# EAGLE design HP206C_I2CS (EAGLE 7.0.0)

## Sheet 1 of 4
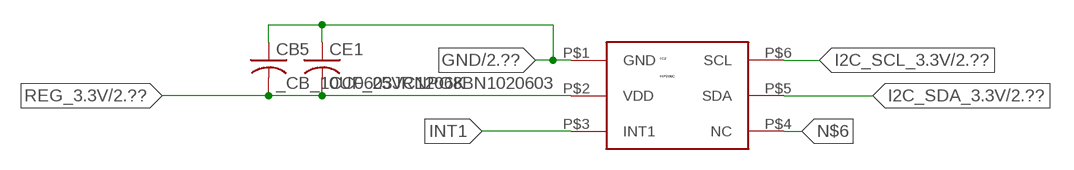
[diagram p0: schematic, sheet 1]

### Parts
CB5  _CB_10UF_25VC1206K  [_CB_10UF_25V]
CE1  CC0603JRNPO8BN1020603  [CC0603JRNPO8BN102]
IC2  HP206C  [HP206C]

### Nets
GND: CB5.1 CE1.1 IC2.P$1(GND) ; also sheet 2,4
I2C_SCL_3.3V: IC2.P$6(SCL) ; also sheet 2
I2C_SDA_3.3V: IC2.P$5(SDA) ; also sheet 2
INT1: IC2.P$3(INT1)
N$6: IC2.P$4(NC)
REG_3.3V: CB5.2 CE1.2 IC2.P$2(VDD) ; also sheet 2

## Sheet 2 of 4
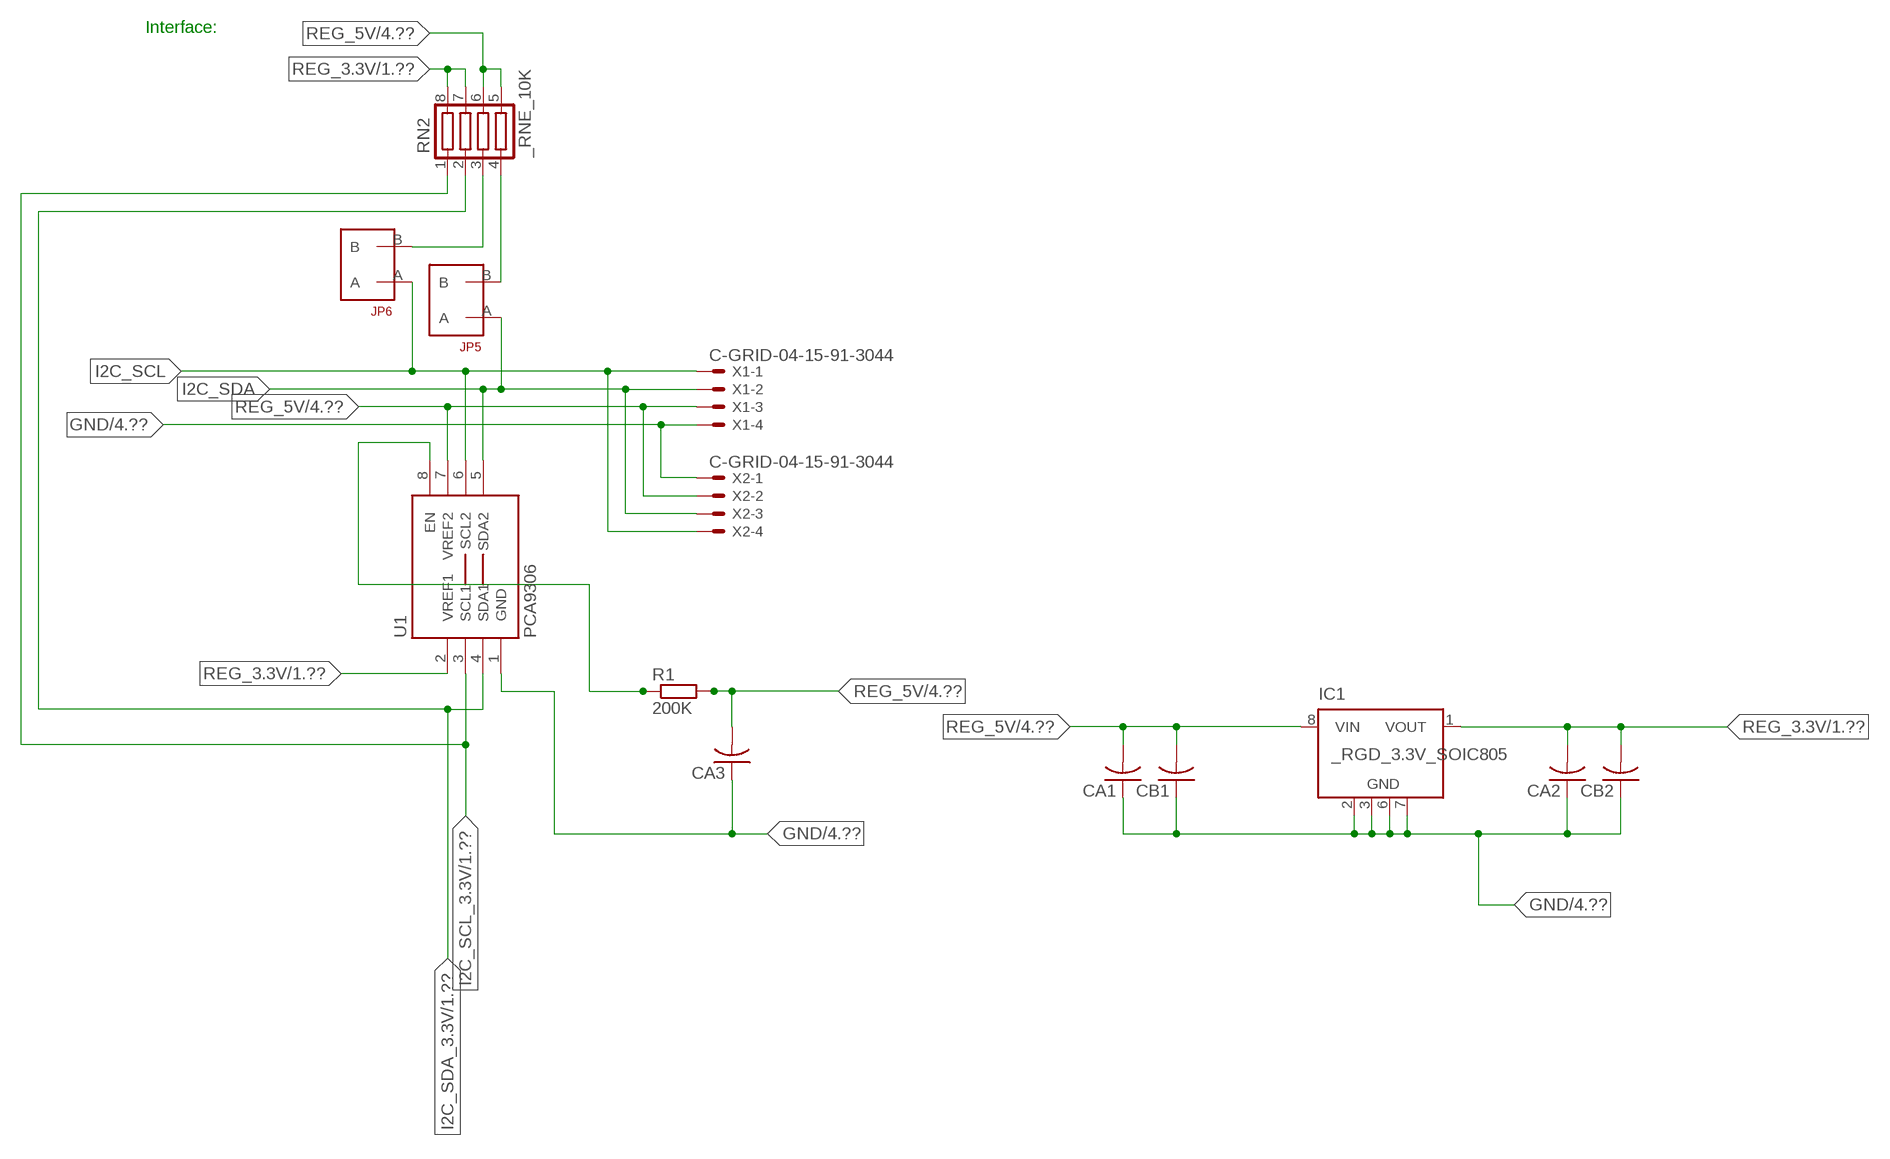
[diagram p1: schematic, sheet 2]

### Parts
CA1  CC1206KRX7R9BB104  [.1UF]
CA2  CC1206KRX7R9BB104  [.1UF]
CA3  CC1206KRX7R9BB104  [.1UF]
CB1  TMK316F106ZL-TC1206K  [TMK316F106ZL-T]
CB2  TMK316F106ZL-TC1206K  [TMK316F106ZL-T]
IC1  _RGD_3.3V_SOIC805  [_RGC_3.3V_SOIC8]
JP5  JUMPER_1X2_2MM  [JUMPER_1X2_2MM]
JP6  JUMPER_1X2_2MM  [JUMPER_1X2_2MM]
R1  200K  RESISTOR_SMT-0603  [R603]
RN2  _RNE_10K  [RNE]
U1  PCA9306  PCA9306_NCD  [PSOP-8]
X1  C-GRID-04-15-91-3044  [15-91-04]
X2  C-GRID-04-15-91-3044  [15-91-04]

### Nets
GND: CA1.1 CA2.1 CA3.1 CB1.1 CB2.1 IC1.2(GND) IC1.3(GND) IC1.6(GND) IC1.7(GND) U1.1(GND) X1.4 X2.1 ; also sheet 1,4
I2C_SCL: JP6.A U1.6(SCL2) X1.1 X2.4
I2C_SCL_3.3V: RN2.1 U1.3(SCL1) ; also sheet 1
I2C_SDA: JP5.A U1.5(SDA2) X1.2 X2.3
I2C_SDA_3.3V: RN2.2 U1.4(SDA1) ; also sheet 1
N$1: JP6.B RN2.3
N$2: JP5.B RN2.4
N$3: R1.1 U1.8(EN)
REG_3.3V: CA2.2 CB2.2 IC1.1(VOUT) RN2.7 RN2.8 U1.2(VREF1) ; also sheet 1
REG_5V: CA1.2 CA3.2 CB1.2 IC1.8(VIN) R1.2 RN2.5 RN2.6 U1.7(VREF2) X1.3 X2.2 ; also sheet 4
Unconnected: IC1.4(NC) IC1.5(NC)

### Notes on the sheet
- Interface:

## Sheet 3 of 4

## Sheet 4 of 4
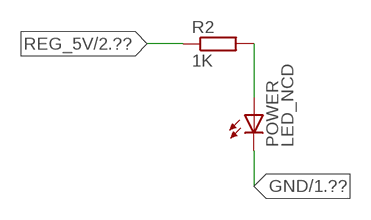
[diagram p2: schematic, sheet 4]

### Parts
POWER  LED_NCD  [CHIPLED_0603]
R2  1K  RESISTOR_SMT-0402  [R402]

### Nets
GND: POWER.C ; also sheet 1,2
N$4: POWER.A R2.2
REG_5V: R2.1 ; also sheet 2

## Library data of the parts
CA1-CA3 = NCD_ULTIMATE_LIBRARY:CC1206KRX7R9BB104: Capacitor CA .1uF 50V SMT C1206K CC1206KRX7R9BB104
CB1 CB2 = NCD_ULTIMATE_LIBRARY:TMK316F106ZL-T: Capacitor CB 10uF SMT 1206 TMK316F106ZL-T
CB5 = NCD_ULTIMATE_LIBRARY:_CB_10UF_25V: Capacitor 10uF SMT
CE1 = NCD_ULTIMATE_LIBRARY:CC0603JRNPO8BN102: Capacitor CE 1uF SMT CC0603JRNPO8BN102 0603
IC1 = NCD_ULTIMATE_LIBRARY:_RGD_3.3V_SOIC8: Regulator Linear 3.3V Chip Positive VOLTAGE REGULATOR Digikey 497-1199-2-ND/L78L33ACD13TR
IC2 = NCD_ULTIMATE_bhaskar:HP206C: Pressue Sensor HP206C http://www.hoperf.com/upload/sensor/HP206C_DataSheet_EN_V2.0.pdf
JP5 JP6 = NCD_ULTIMATE_CONNECTORS:JUMPER_1X2_2MM
POWER = NCD_ULTIMATE_LIBRARY:LED_NCD: LED Digikey 754-1132-2-ND/APT2012SRCPRV
R1 R2 = NCD_ULTIMATE_LIBRARY:RESISTOR_SMT: NCD Resistor
RN2 = NCD_ULTIMATE_LIBRARY:_RNE_10K: Resistor Array RNE SMT 10K x 4 Single Resistor Source: http://www.ctscorp.com/components/Datasheets/CTSChipArrayDs.pdf Digikey 742C083103JPTR-ND/742C083103JP; OC_FARNELL: unknown; OC_NEWARK: unknown
U1 = NCD_ULTIMATE_LIBRARY:PCA9306_NCD: NCD Bidirectional I2C level shifter. NOT compatible with all available part number pinout schemes- DOUBLE CHECK!!!; PROD_ID: IC-10023
X1 X2 = NCD_ULTIMATE_CONNECTORS:C-GRID-04: CONNECTOR 4-Pos I2C wire to board 2.54 mm (0.100") pitch header Digikey WM1342-ND/0015912045; OC_FARNELL: unknown; OC_NEWARK: unknown

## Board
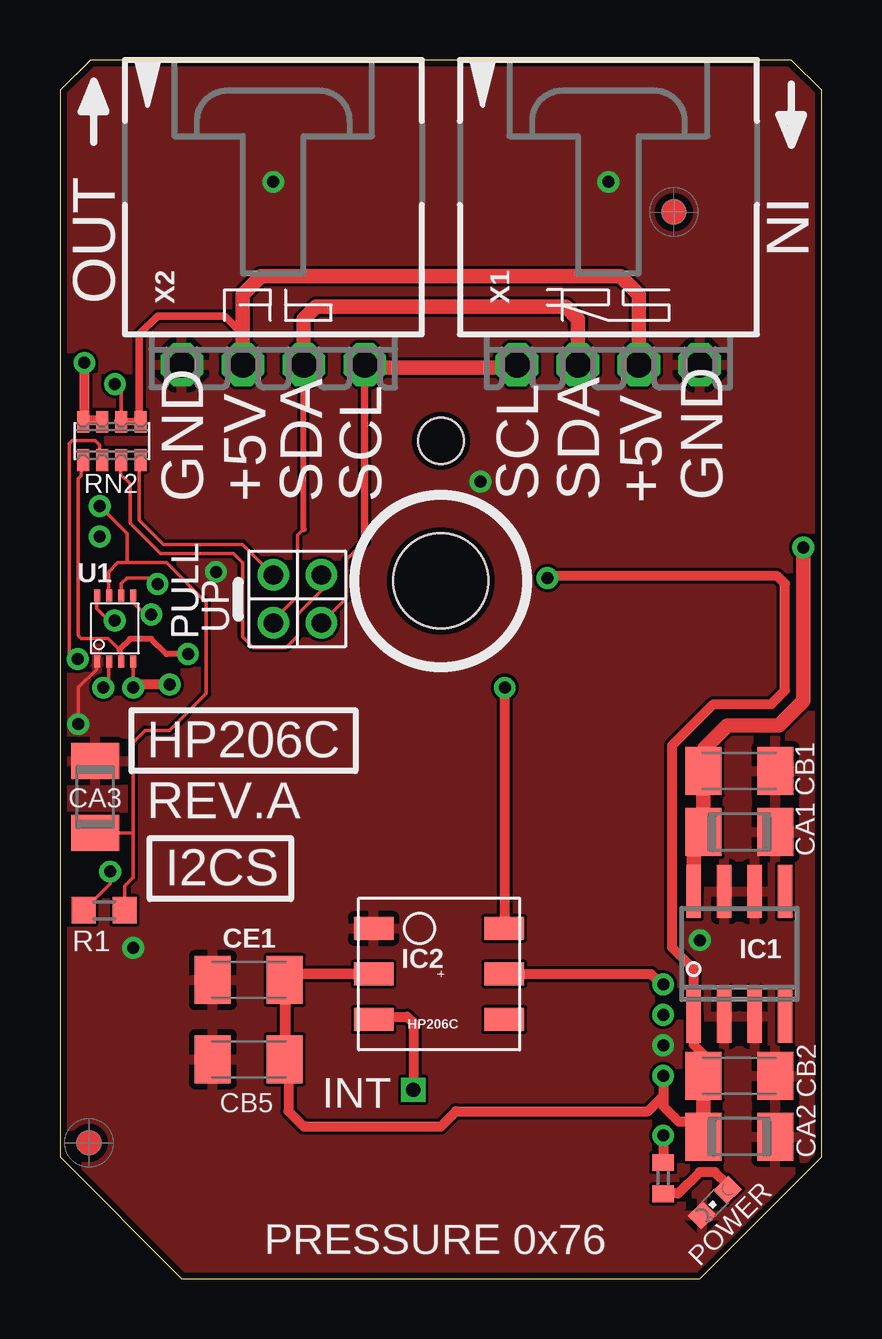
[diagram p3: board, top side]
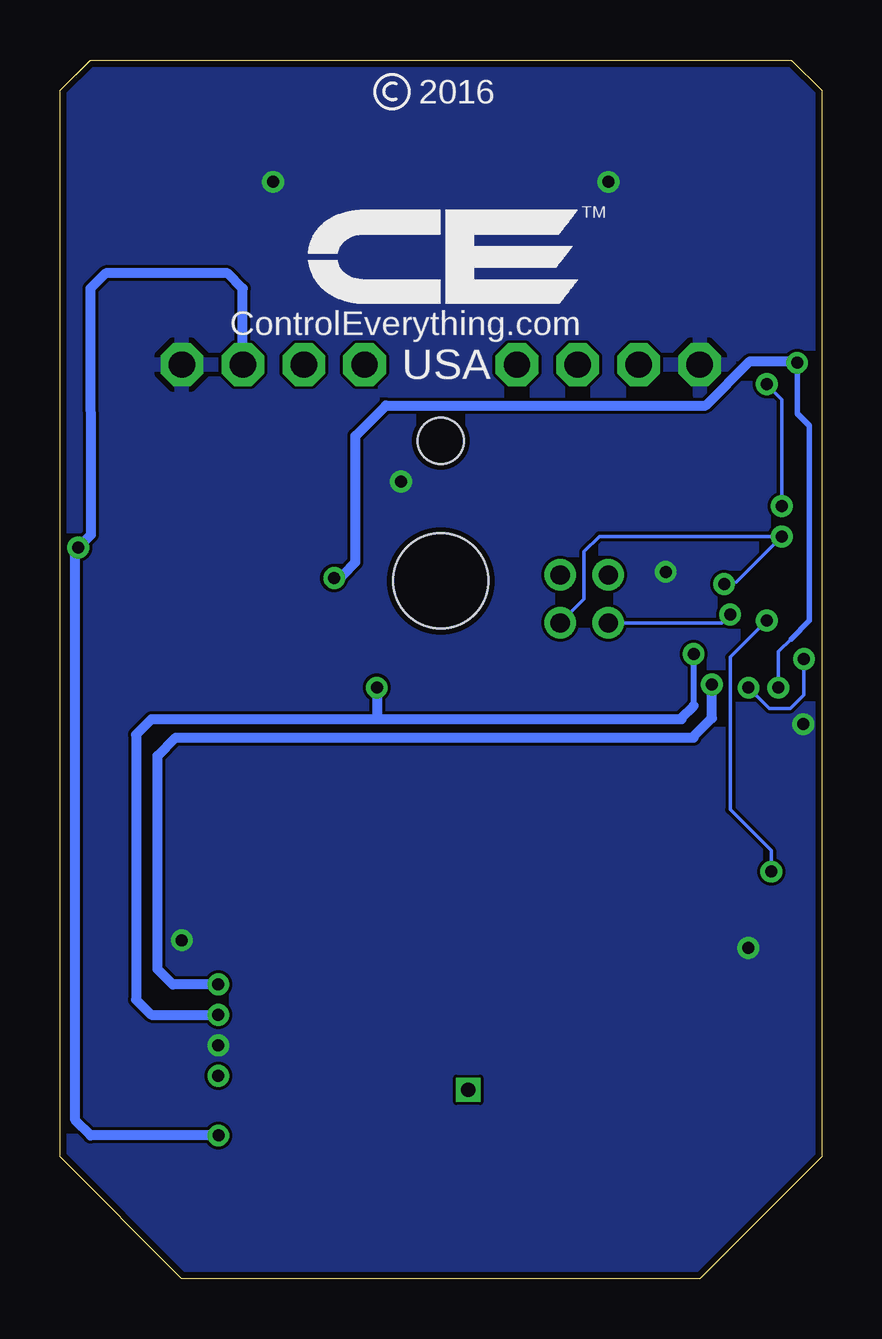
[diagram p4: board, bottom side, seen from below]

Size 31.75 x 50.8 mm. Coordinates in mm from the lower left corner, seen from the top.
Outline: 32 segments
Copper layers (1*16): Top 0.035mm / dielectric 1.5mm / Bottom 0.035mm
Design rules "default": minimum track width 5mil, minimum drill 24mil, track to track 5mil, track to pad 5mil, pad to pad 5mil, via to via 5mil, smd to smd 5mil, copper to edge 10mil, drill to drill 8mil, minimum pad ring 10mil, minimum via ring 8mil, stop-mask expansion 2mil, vias tented up to drill 0mil, thermal gap 10mil
Holes 3.96 mm at 15.88,29.08 15.88,29.08
Holes 1.91 mm at 15.88,34.93 15.88,34.93

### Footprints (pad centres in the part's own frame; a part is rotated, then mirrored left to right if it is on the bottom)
.1UF = smd 1.5 x 2: 1 -1.5,0; 2 1.5,0
TMK316F106ZL-T = smd 1.5 x 2: 1 -1.5,0; 2 1.5,0
_CB_10UF_25V = smd 1.5 x 2: 1 -1.5,0; 2 1.5,0
CC0603JRNPO8BN102 = smd 1.5 x 2: 1 -1.5,0; 2 1.5,0
_RGC_3.3V_SOIC8 = smd 0.6 x 2.2: 1 -1.905,-2.6; 2 -0.635,-2.6; 3 0.635,-2.6; 4 1.905,-2.6; 5 1.905,2.6; 6 0.635,2.6; 7 -0.635,2.6; 8 -1.905,2.6
HP206C = smd 1.65 x 0.95: P$1 -1.905,1.905; P$2 -1.905,0.005; P$3 -1.905,-1.895; P$4 3.536,-1.895; P$5 3.536,0.005; P$6 3.536,1.905
JUMPER_1X2_2MM = drill 0.8: A 0,2; B 0,0
CHIPLED_0603 = smd 0.8 x 0.876: A 0,-0.75; C 0,0.75
R603 = smd 1 x 1.1: 1 -0.85,0; 2 0.85,0
R402 = smd 0.7 x 0.9: 1 -0.65,0; 2 0.65,0
RNE = smd 0.5 x 0.9: 1 -1.2,-0.8; 2 -0.4,-0.8; 3 0.4,-0.8; 4 1.2,-0.8; 5 1.2,0.8; 6 0.4,0.8; 7 -0.4,0.8; 8 -1.2,0.8
PSOP-8 = smd 0.25 x 0.5: 1 -0.73,-1.37; 2 -0.23,-1.37; 3 0.27,-1.37; 4 0.77,-1.37; 5 0.77,1.38; 6 0.27,1.38; 7 -0.23,1.38; 8 -0.73,1.38
15-91-04 = drill 1.1 pad 1.778 octagon: 1 -3.81,-7.62; 2 -1.27,-7.62; 3 1.27,-7.62; 4 3.81,-7.62

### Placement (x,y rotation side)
CA1  28.32,18.62 180 top
CA2  28.32,5.92 180 top
CA3  1.46,20.08 270 top
CB1  28.32,21.16 180 top
CB2  28.32,8.46 180 top
CB5  7.87,9.14 0 top
CE1  7.87,12.45 0 top
IC1  28.32,13.54 0 top
IC2  14.99,12.7 0 top
JP5  8.89,29.34 180 top
JP6  10.9,29.34 180 top
POWER  27.3,3.18 135 top
R1  1.84,15.35 0 top
R2  25.15,4.19 270 top
RN2  2.16,34.93 0 top
U1  2.28,27.1 0 top
U$5  [VISION_REF10]  1.21,5.66 90 top
U$28  [VISION_REF10]  25.59,44.46 90 top
X1  22.86,45.72 0 top
X2  8.89,45.72 0 top

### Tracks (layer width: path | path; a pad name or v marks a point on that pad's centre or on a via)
GND  (via drill 0.5)
  Top 0.152: CA3.1 1.52,21.64 1.52,21.59 | U1.1 1.52,25.7 1.52,25.4 0.76,24.64 v0.76,23.11
  other vias: 8.89,45.72 22.86,45.72 25.15,9.73 17.53,33.22 26.67,14.11 3.05,13.79 8.89,45.72 22.86,45.72 25.15,9.73 17.53,33.22 6.5,29.46
  pour Top: -1.27,0 -1.27,50.8 33.02,50.8 33.02,0
  pour Bottom: -5.08,0 -5.08,50.8 35.56,50.8 35.56,0
I2C_SCL  (via drill 0.5)
  Top 0.152: 12.7,30.73 11.94,29.97 11.94,28.38 JP6.A | v4.06,28.96 3.81,29.21 2.79,29.21 2.55,28.97 U1.6
  Top 0.305: 12.7,30.73 X2.4
  Top 0.406: X2.4 12.7,37.97 | 19.05,37.97 X1.1
  Top 0.61: 12.7,37.97 19.05,37.97
  Bottom 0.152: JP6.A 9.91,28.33 9.91,30.3 9.27,30.94 v1.65,30.94 3.56,29.04 v4.06,28.96
I2C_SCL_3.3V  (via drill 0.5)
  Top 0.152: RN2.1 0.89,34.07 0.89,33.48 0.77,33.35 0.77,26.81 0.89,26.68 2.02,26.68 2.48,26.23 2.55,26.15 U1.3
  Top 0.254: v5.33,26.04 4.45,26.04 3.81,26.67 2.92,26.67 2.48,26.23
  Top 0.406: IC2.P$6 18.54,15.47 v18.54,24.64
  Bottom 0.254: 5.33,23.88 v5.33,26.04
  Bottom 0.406: 18.54,23.32 5.84,23.32 5.84,23.37 5.33,23.88 | 18.54,23.32 27.94,23.32 28.58,22.68 28.58,11.63 27.94,11 v25.15,11 | v18.54,24.64 18.54,23.32
I2C_SDA  (via drill 0.5)
  Top 0.152: JP5.A 8.89,27.44 9.91,28.45 9.91,30.99 10.16,31.24 | U1.5 3.05,28.19 3.56,27.69 v3.81,27.69
  Top 0.254: 10.16,31.24 10.16,31.25 X2.3
  Top 0.61: X2.3 10.16,40.01 10.67,40.51 21.09,40.51 21.59,40.01 X1.2
  Bottom 0.152: v3.81,27.69 4.16,27.34 JP5.A
I2C_SDA_3.3V  (via drill 0.5)
  Top 0.152: RN2.2 1.65,34.14 1.65,34.75 1.46,34.94 0.51,34.94 0.38,34.81 0.38,25.78 v0.74,25.83 | U1.4 v3.05,24.64
  Top 0.406: IC2.P$5 18.78,12.7 24.64,12.7 25.07,12.27 v25.15,12.27 | v4.57,24.77 3.17,24.77 v3.05,24.64
  Bottom 0.152: v3.05,24.64 2.18,23.77 1.29,23.77 0.74,24.33 v0.74,25.83
  Bottom 0.406: v25.15,12.27 27.05,12.27 27.69,12.9 27.69,21.79 26.93,22.56 5.34,22.56 5.34,22.6 4.57,23.37 v4.57,24.77
INT1  (via drill 0.6)
  Top 0.406: IC2.P$3 13.45,10.92 14.48,10.92 14.73,10.67 v14.73,7.87
N$1
  Top 0.152: JP6.B 10.92,29.31 10.92,28.7 9.91,27.69 9.91,26.8 9.42,26.31 8.06,26.31 7.62,26.75 7.62,29.84 7.24,30.23 4.19,30.23 2.92,31.5 2.92,33.15 2.54,33.53 2.54,34.1 RN2.3
  Top 0.305: 2.54,34.02 RN2.3
N$2
  Top 0.152: JP5.B 7.62,30.61 4.32,30.61 3.3,31.62 3.3,34.07 RN2.4
  Top 0.305: 3.37,33.88 RN2.4
N$3  (via drill 0.5)
  Top 0.152: R1.1 2.1,16.46 v2.1,16.97 | U1.8 1.52,28.45 1.52,27.94 2.03,27.43 v2.29,27.43
  Bottom 0.152: v2.29,27.43 3.81,25.91 3.81,19.56 2.1,17.85 v2.1,16.97
N$4
  Top 0.406: POWER.A 27.84,3.92 27.3,4.45 26.67,4.45 25.78,3.56 25.16,3.56 R2.2
REG_3.3V  (via drill 0.5)
  Top 0.152: v1.8,24.64 1.8,24.91 | v1.8,24.64 2.03,24.64 2.03,25.65 2.05,25.68 U1.2 | 1.78,24.64 v1.8,24.64
  Top 0.406: 26.67,6.55 26.82,6.55 | 26.67,5.33 26.67,6.55 | 9.65,8.89 9.4,9.14 9.4,12.7 13.33,12.7 IC2.P$2 9.63,12.71 CE1.2 CB5.2 9.53,8.99 9.53,6.99 10.16,6.35 15.88,6.35 16.51,6.99 24.51,6.99 25.15,7.62 | CB2.2 26.82,9.35 26.42,9.75 26.42,10.36 | v25.15,8.46 25.15,7.62 | 25.15,7.62 25.15,7.19 25.78,6.55 26.67,6.55 | IC1.1 26.42,12.9 25.53,13.79 25.53,22.24 27.24,23.95 29.66,23.95 30.23,24.52 30.23,28.97 29.91,29.29 20.4,29.29 v20.32,29.21 | 26.52,5.62 CA2.2 | v1.02,38.18 1.02,35.78 | 1.02,35.78 RN2.8 | 1.02,35.78 1.71,35.78 RN2.7
  Top 0.61: CB2.2 26.82,6.55 CA2.2 | 26.42,10.36 IC1.1
  Bottom 0.152: 1.27,26.67 1.8,26.14 v1.8,24.64
  Bottom 0.229: 1.27,26.67 0.51,27.43 0.51,35.56 1.02,36.07 v1.02,38.18
  Bottom 0.406: v1.02,38.18 1.08,38.24 2.99,38.24 4.83,36.4 18.16,36.4 19.43,35.13 19.43,29.87 19.94,29.34 20.07,29.21 v20.32,29.21
REG_5V  (via drill 0.5)
  Top 0.152: RN2.6 2.56,37.01 v2.29,37.29 | 3.05,18.58 3.05,16.73 2.69,16.37 R1.2 | 3.05,18.58 3.05,22.35 3.56,22.86 4.57,22.86 6.1,24.38 6.1,28.19 4.45,29.85 2.79,29.85 | CA3.2 3.05,18.58 | v1.65,32.21 2.79,31.07 2.79,29.85 | 2.79,29.85 2.41,29.85 2.03,29.46 2.03,28.5 U1.7
  Top 0.305: 7.62,39.37 7.5,39.37 | 2.42,35.74 RN2.6 RN2.5 3.31,35.8 3.31,39.37 4.07,40.13 6.86,40.13 7.62,39.37 | X2.2 7.62,39.37
  Top 0.406: v25.15,5.97 R2.1
  Top 0.61: X2.2 7.62,41.02 8.38,41.78 23.37,41.78 24.13,41.02 X1.3 | IC1.8 26.42,18.21 CA1.2 CB1.2 26.86,21.2 26.86,22.11 27.82,23.06 29.98,23.06 30.99,24.08 v30.99,30.48
  Bottom 0.152: v1.65,32.21 1.65,36.65 v2.29,37.29
  Bottom 0.406: X1.3 24.13,41.28 24.77,41.91 29.84,41.91 30.48,41.27 30.47,31 v30.99,30.48 31.11,30.36 31.11,6.6 30.48,5.97 v25.15,5.97

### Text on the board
tNames: IN | IN | OUT | OUT | GND | +5V | SDA | SCL | SCL | SDA | +5V | GND | PULL | PULL | UP | UP | HP206C | REV.A | I2CS | INT | PRESSURE 0x76
bNames: 2016 | TM | ControlEverything.com | USA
